DATA_BLOCK DB 4
VERSION : 0.1


  STRUCT
   SEN_REC_SFC65 : BOOL ;
   SEN_REC_SFC651 : BOOL ;
   SEN_REC_SFC652 : BOOL ;
   SEN_REC_SFC653 : BOOL ;
   SEN_REC_SFC654 : BOOL ;
   SEN_REC_SFC655 : BOOL ;
   SEN_REC_SFC656 : BOOL ;
   SEN_REC_SFC657 : BOOL ;
   SEN_REC_SFC658 : BOOL ;
   SEN_REC_SFC659 : BOOL ;
   SEN_REC_SFC6510 : BOOL ;
   SEN_REC_SFC6511 : BOOL ;
   SEN_REC_SFC6512 : BOOL ;
   SEN_REC_SFC6513 : BOOL ;
   SEN_REC_SFC6514 : BOOL ;
   SEN_REC_SFC6515 : BOOL ;
   SEN_REC_RETVAL : INT ;
   SEN_REC_VALUE : DWORD ;
   SEN_REC_DATA : DWORD ;
  END_STRUCT ;
BEGIN
   SEN_REC_SFC65 := FALSE;
   SEN_REC_SFC651 := FALSE;
   SEN_REC_SFC652 := FALSE;
   SEN_REC_SFC653 := FALSE;
   SEN_REC_SFC654 := FALSE;
   SEN_REC_SFC655 := FALSE;
   SEN_REC_SFC656 := FALSE;
   SEN_REC_SFC657 := FALSE;
   SEN_REC_SFC658 := FALSE;
   SEN_REC_SFC659 := FALSE;
   SEN_REC_SFC6510 := FALSE;
   SEN_REC_SFC6511 := FALSE;
   SEN_REC_SFC6512 := FALSE;
   SEN_REC_SFC6513 := FALSE;
   SEN_REC_SFC6514 := FALSE;
   SEN_REC_SFC6515 := FALSE;
   SEN_REC_RETVAL := 0;
   SEN_REC_VALUE := DW#16#0;
   SEN_REC_DATA := DW#16#0;
END_DATA_BLOCK

